TYPE E_PMLState : (
(* states according to PackTags v3.0 *)
	ePMLState_UNDEFINED		:=  0,
	ePMLState_CLEARING 		:=  1,
	ePMLState_STOPPED 		:=  2,
	ePMLState_STARTING 		:=  3,
	ePMLState_IDLE 			:=  4,
	ePMLState_SUSPENDED 	:=  5,
	ePMLState_EXECUTE 		:=  6,
	ePMLState_STOPPING	 	:=  7,
	ePMLState_ABORTING 		:=  8,
	ePMLState_ABORTED 		:=  9,
	ePMLState_HOLDING 		:= 10,
	ePMLState_HELD 			:= 11,
	ePMLState_UNHOLDING 	:= 12,
	ePMLState_SUSPENDING 	:= 13,
	ePMLState_UNSUSPENDING 	:= 14,
	ePMLState_RESETTING 	:= 15,
	ePMLState_COMPLETING 	:= 16,
	ePMLState_COMPLETE	 	:= 17
);
END_TYPE
